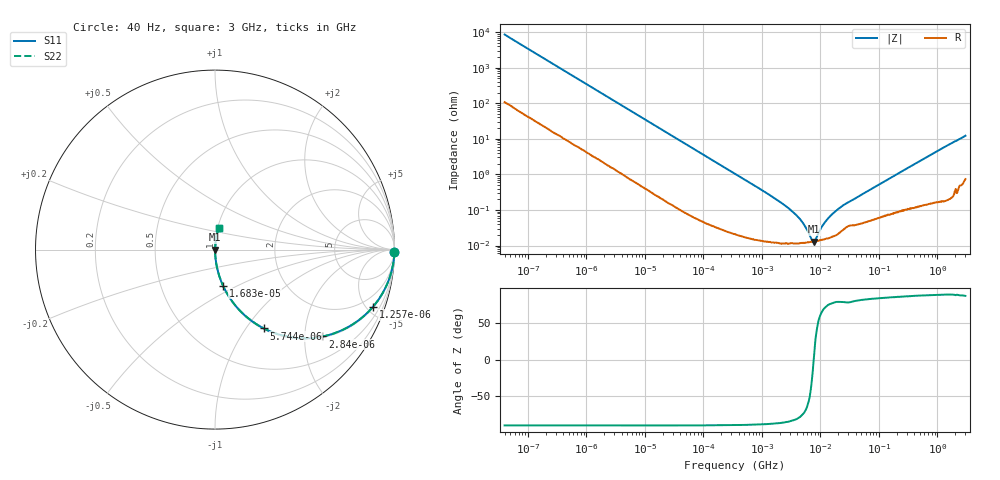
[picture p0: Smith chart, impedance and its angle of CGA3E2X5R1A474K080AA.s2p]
! S-parameter Generated by TDK Corporation
! Copyright(C) 2015 TDK Corporation.
! All Rights Reserved.
! TDK P/N: CGA3E2X5R1A474K080AA (Multilayer Ceramic Chip Capacitors)
! Property: C=470nF
! Size(LxWxT): 1.6x0.8x0.8mm, 0.063x0.031x0.031inches
! Model Type: s2p (Touchstone File Format Version 1.0)
! Frequency: DC=Yes Start=0.00004MHz Stop=3000MHz 568points Log-sweep
! Note: This model was converted from impedance.
! Model Generated on Jun. 23, 2015
! Hash(MD5):
! Port Assignments:
!  1 ---| |--- 2
! Applicable Conditions:
!  Temperature = 25 degC
!  DC Bias Voltage = 0 V
!  Small Signal Operation
! Terms and conditions regarding TDK Simulation Models
! (1)This simulation model is being provided solely for informational purposes. Please refer to the specifications of the products in terms of detailed characteristics of such products.
! (2)In no event shall TDK Corporation of any of its subsidiaries be liable for any loss or damage arising, directly or indirectly,
!  From any information contained in this simulation model, including, but not limited to loss or damages arising from any inaccuracies, omissions or errors in connection with such information.
! (3)Any and all copyrights on this simulation model are owned by TDK Corporation.
!  Duplication or redistribution of this simulation model without prior written permission from TDK Corporation is prohibited.
! (4)This simulation model is subject to any modification or change without any prior notice.
! (5)Neither TDK Corporation nor any of its subsidiaries shall make any warranty, express or implied,
!  Including but not limited to the correctness, implied warranties of merchantability and fitness for a particular purpose with respect to this simulation models.
! (6)The use of this simulation model shall be deemed to have consented to the terms and conditions hereof.
# MHz S MA R 50
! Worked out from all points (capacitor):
!   567 points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, 40 Hz to 3 GHz, reference 50 ohm
!   read as one part in series: C = 469 nF near 43.08 Hz
!   lowest |Z| = 12.8 mohm at 7.626 MHz (marker M1)
!   series resonance near 7.673 MHz, so ESL is about 920 pH
!   S11 on the Smith chart (normalised r, x): 40 Hz: open; 1.257 kHz: 1.07, -5.51; 2.84 kHz: 1.03, -2.45; 5.744 kHz: 1.01, -1.22; 16.83 kHz: 1.00, -0.42; 3 GHz: 1.01, +0.24
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4e-05  0.9998 -0.7  0.01167 88.6  0.01167 88.6  0.9998 -0.7
0.000245968  0.9966 -4.1  0.07161 85.2  0.07161 85.2  0.9966 -4.1
0.00083584  0.9692 -13.6  0.2348 75.7  0.2348 75.7  0.9692 -13.6
0.001256623  0.9363 -19.9  0.3401 69.4  0.3401 69.4  0.9363 -19.9
0.002840326  0.77 -39.0  0.6288 50.3  0.6288 50.3  0.77 -39.0
0.005744291  0.5173 -58.2  0.8498 31.1  0.8498 31.1  0.5173 -58.2
0.009300681  0.3519 -68.7  0.932 20.6  0.932 20.6  0.3519 -68.7
0.01683015  0.2051 -77.5  0.9764 11.8  0.9764 11.8  0.2051 -77.5
0.01746572  0.198 -77.9  0.978 11.4  0.978 11.4  0.198 -77.9
0.0571917  0.06259 -85.8  0.9973 3.6  0.9973 3.6  0.06259 -85.8
0.3516829  0.01035 -88.3  0.9997 0.6  0.9997 0.6  0.01035 -88.3
1.607618  0.002192 -86.7  0.9999 0.1  0.9999 0.1  0.002192 -86.7
3.132945  0.0009848 -83.1  0.9999 0.1  0.9999 0.1  0.0009848 -83.1
4.888018  0.0004607 -75.1  0.9999 0.0  0.9999 0.0  0.0004607 -75.1
7.348767  0.0001335 -17.6  0.9999 0.0  0.9999 0.0  0.0001335 -17.6
7.626281  0.0001284 -2.7  0.9999 0.0  0.9999 0.0  0.0001284 -2.7
8.213145  0.0001482 27.4  0.9999 -0.0  0.9999 -0.0  0.0001482 27.4
11.89852  0.0004506 70.3  0.9998 -0.0  0.9998 -0.0  0.0004506 70.3
19.26509  0.001008 78.3  0.9998 -0.1  0.9998 -0.1  0.001008 78.3
149.005  0.007545 84.0  0.9992 -0.4  0.9992 -0.4  0.007545 84.0
867.2962  0.04007 85.4  0.9976 -2.3  0.9976 -2.3  0.04007 85.4
3000  0.1203 79.6  0.9855 -6.9  0.9855 -6.9  0.1203 79.6
